| TEXAS INSTRUMENTS INCORPORATED
| Standard Linear and Logic Group
| IBIS Model of SN74CBTLV3253
| LOW-VOLTAGE DUAL 1-OF-4 FET MULTIPLEXER/DEMULTIPLEXER
| This file contains package information for the following:
|  SOIC 16-pin (D) package as [Component] CBTLV3253_D
|  TSSOP 16-pin (PW) package as [Component] CBTLV3253_PW
|  SSOP 16-pin (DBQR) package as [Component] CBTLV3253_DBQR
|  TVSOP 16-pin (DGV) package as [Component] CBTLV3253_DGV
|  QFN 16-pin (RGY) package as [Component] CBTLV3253_RGY
| This device can be powered at the following Vccs:
|  3.3 volt Vcc
|  2.5 volt Vcc
| This file provides unique models under the [Model Selector] for each Vcc.
| For operation at a specific Vcc, select the appropriate model after each
| [Model Selector] keyword.
[IBIS Ver]   3.2
[Comment char]  |_char
[File Name]   sn74cbtlv3253.ibs
[File Rev]   1.1 | x_die
[Date]   August 14, 2003
[Source]   Data created from TI-SPICE simulations at TI-SLL.
[Notes]   The following is an IBIS list for the CBTLV3253.
   Please contact sllibis@ti.com with questions and
   comments concerning SLL IBIS models.
   - The terminator models are for A-port only.
   - C_comp values have been replaced by the data sheet values in
   the terminator models.
   - Power clamp data deleted as there is no power-clamp diode.
   - Non-monotonic data due to FET characteristics.
[Disclaimer] Property of Texas Instruments Incorporated.  Unauthorized
   reproduction and/or distribution is strictly prohibited.
   This product is protected under copyright law.
   Created  2003, (C) Copyright  2003, Texas Instruments
   Incorporated, All Rights Reserved
   UNLESS THERE IS A SIGNED, WRITTEN AGREEMENT TO THE
   CONTRARY, TEXAS INSTRUMENTS (TI) IS PROVIDING THE IBIS
   MODELS  AND WITHOUT ANY WARRANTY, EXPRESSED OR
   IMPLIED.  TI assumes no liability for:
   1) the accuracy of the IBIS models provided to your
   company;
   2) the proper functioning of these IBIS Models in your
   design or for any resulting applications; or
   3) infringement of patents, copyrights or intellectual
   property rights resulting from your use of these IBIS
   models.
   TI provides IBIS Models as a service to our customers.
   You and your company shall not distribute, sell or give
   these models to anyone else without prior written
   permission from TI.
   TI reserves the right to make changes to our products or
   to discontinue any semiconductor product or service
   without notice, and advises our customers to obtain the
   latest version of relevant information to verify, before
   placing orders, that the information being relied on is
   current.
   Please be aware that your receipt and use of the IBIS
   information provided shall serve as acceptance of these
   terms and conditions.  If you do not accept these terms,
   you should return or destroy the IBIS models and any
   other accompanying information immediately.
| Component CBTLV3253_D 16-pin SOIC
[Component]   CBTLV3253_D
[Manufacturer]   Texas Instruments, Inc.
[Package]
|   typ   min   max
R_pkg   3.900e-02   2.800e-02   4.900e-02
L_pkg   3.453e-09   2.350e-09   4.375e-09
C_pkg   5.210e-13   2.540e-13   7.080e-13
[Pin]   signal_name   model_name   R_pin   L_pin   C_pin
1   1NOE   CBTLV3253_NOE   4.200e-02   4.336e-09   7.030e-13
2   S1   CBTLV3253_IN   4.900e-02   3.778e-09   6.340e-13
3   1B4   CBTLV3253_IO   2.800e-02   3.449e-09   5.180e-13
4   1B3   CBTLV3253_IO   2.900e-02   2.393e-09   2.540e-13
5   1B2   CBTLV3253_IO   2.800e-02   2.350e-09   2.640e-13
6   1B1   CBTLV3253_IO   4.800e-02   3.312e-09   4.830e-13
7   1A   CBTLV3253_IO   4.300e-02   3.629e-09   6.040e-13
8   GND   GND   4.400e-02   4.375e-09   7.080e-13
9   2A   CBTLV3253_IO   4.200e-02   4.336e-09   7.030e-13
10   2B1   CBTLV3253_IO   4.900e-02   3.778e-09   6.340e-13
11   2B2   CBTLV3253_IO   2.800e-02   3.449e-09   5.180e-13
12   2B3   CBTLV3253_IO   2.900e-02   2.393e-09   2.550e-13
13   2B4   CBTLV3253_IO   2.800e-02   2.350e-09   2.640e-13
14   S0   CBTLV3253_IN   4.800e-02   3.312e-09   4.830e-13
15   2NOE   CBTLV3253_NOE   4.300e-02   3.629e-09   6.040e-13
16   VCC   POWER   4.400e-02   4.375e-09   7.080e-13
| Component CBTLV3253_PW 16-pin TSSOP
[Component]   CBTLV3253_PW
[Manufacturer]   Texas Instruments, Inc.
[Package]
|   typ   min   max
R_pkg   4.500e-02   3.800e-02   5.100e-02
L_pkg   2.593e-09   2.447e-09   3.080e-09
C_pkg   2.810e-13   2.430e-13   3.770e-13
[Pin]   signal_name   model_name   R_pin   L_pin   C_pin
1   1NOE   CBTLV3253_NOE   4.000e-02   3.080e-09   3.770e-13
2   S1   CBTLV3253_IN   3.800e-02   2.458e-09   2.810e-13
3   1B4   CBTLV3253_IO   5.100e-02   2.512e-09   2.550e-13
4   1B3   CBTLV3253_IO   5.100e-02   2.447e-09   2.430e-13
5   1B2   CBTLV3253_IO   5.100e-02   2.447e-09   2.430e-13
6   1B1   CBTLV3253_IO   5.100e-02   2.512e-09   2.550e-13
7   1A   CBTLV3253_IO   3.800e-02   2.458e-09   2.810e-13
8   GND   GND   4.000e-02   3.080e-09   3.770e-13
9   2A   CBTLV3253_IO   3.900e-02   2.832e-09   3.160e-13
10   2B1   CBTLV3253_IO   3.800e-02   2.460e-09   2.790e-13
11   2B2   CBTLV3253_IO   5.100e-02   2.512e-09   2.550e-13
12   2B3   CBTLV3253_IO   5.100e-02   2.447e-09   2.430e-13
13   2B4   CBTLV3253_IO   5.100e-02   2.447e-09   2.430e-13
14   S0   CBTLV3253_IN   5.100e-02   2.512e-09   2.550e-13
15   2NOE   CBTLV3253_NOE   3.800e-02   2.459e-09   2.790e-13
16   VCC   POWER   3.900e-02   2.832e-09   3.160e-13
| Component CBTLV3253_DBQR 16-pin SSOP
[Component]   CBTLV3253_DBQR
[Manufacturer]   Texas Instruments, Inc.
[Package]
|   typ   min   max
R_pkg   3.800e-02   2.700e-02   5.900e-02
L_pkg   2.353e-09   1.491e-09   4.500e-09
C_pkg   2.100e-13   6.400e-14   5.920e-13
[Pin]   signal_name   model_name   R_pin   L_pin   C_pin
1   1NOE   CBTLV3253_NOE   5.800e-02   4.450e-09   5.920e-13
2   S1   CBTLV3253_IN   4.000e-02   1.930e-09   1.110e-13
3   1B4   CBTLV3253_IO   2.800e-02   1.538e-09   7.600e-14
4   1B3   CBTLV3253_IO   2.700e-02   1.491e-09   6.400e-14
5   1B2   CBTLV3253_IO   2.700e-02   1.491e-09   6.400e-14
6   1B1   CBTLV3253_IO   2.700e-02   1.506e-09   7.500e-14
7   1A   CBTLV3253_IO   3.300e-02   1.922e-09   1.090e-13
8   GND   GND   5.900e-02   4.500e-09   5.880e-13
9   2A   CBTLV3253_IO   5.800e-02   3.695e-09   4.140e-13
10   2B1   CBTLV3253_IO   3.400e-02   2.685e-09   2.820e-13
11   2B2   CBTLV3253_IO   2.900e-02   1.552e-09   7.700e-14
12   2B3   CBTLV3253_IO   2.800e-02   1.506e-09   6.500e-14
13   2B4   CBTLV3253_IO   2.700e-02   1.492e-09   6.400e-14
14   S0   CBTLV3253_IN   2.800e-02   1.534e-09   7.600e-14
15   2NOE   CBTLV3253_NOE   4.000e-02   2.703e-09   2.840e-13
16   VCC   POWER   5.600e-02   3.645e-09   4.180e-13
| Component CBTLV3253_DGV 16-pin TVSOP
[Component]   CBTLV3253_DGV
[Manufacturer]   Texas Instruments, Inc.
[Package]
|   typ   min   max
R_pkg   3.900e-02   3.300e-02   4.500e-02
L_pkg   2.543e-09   2.320e-09   2.938e-09
C_pkg   3.860e-13   3.340e-13   4.490e-13
[Pin]   signal_name   model_name   R_pin   L_pin   C_pin
1   1NOE   CBTLV3253_NOE   3.500e-02   2.907e-09   4.170e-13
2   S1   CBTLV3253_IN   4.200e-02   2.558e-09   4.460e-13
3   1B4   CBTLV3253_IO   3.800e-02   2.341e-09   3.450e-13
4   1B3   CBTLV3253_IO   3.800e-02   2.320e-09   3.340e-13
5   1B2   CBTLV3253_IO   3.900e-02   2.322e-09   3.340e-13
6   1B1   CBTLV3253_IO   3.800e-02   2.353e-09   3.420e-13
7   1A   CBTLV3253_IO   4.000e-02   2.536e-09   4.410e-13
8   GND   GND   3.300e-02   2.897e-09   4.180e-13
9   2A   CBTLV3253_IO   3.500e-02   2.927e-09   4.190e-13
10   2B1   CBTLV3253_IO   4.500e-02   2.632e-09   4.490e-13
11   2B2   CBTLV3253_IO   3.900e-02   2.368e-09   3.470e-13
12   2B3   CBTLV3253_IO   3.900e-02   2.330e-09   3.350e-13
13   2B4   CBTLV3253_IO   3.900e-02   2.320e-09   3.350e-13
14   S0   CBTLV3253_IN   3.900e-02   2.361e-09   3.450e-13
15   2NOE   CBTLV3253_NOE   4.100e-02   2.573e-09   4.460e-13
16   VCC   POWER   3.500e-02   2.938e-09   4.200e-13
| Component CBTLV3253_RGY 16-pin QFN
[Component]   CBTLV3253_RGY
[Manufacturer]   Texas Instruments, Inc.
[Package]
|   typ   min   max
R_pkg   3.000e-02   2.700e-02   3.800e-02
L_pkg   8.000e-10   7.220e-10   9.400e-10
C_pkg   1.410e-13   1.290e-13   1.550e-13
[Pin]   signal_name   model_name   R_pin   L_pin   C_pin
1   1NOE   CBTLV3253_NOE   2.700e-02   8.180e-10   1.320e-13
2   S1   CBTLV3253_IN   2.700e-02   8.030e-10   1.300e-13
3   1B4   CBTLV3253_IO   3.700e-02   9.080e-10   1.500e-13
4   1B3   CBTLV3253_IO   2.900e-02   7.220e-10   1.390e-13
5   1B2   CBTLV3253_IO   2.900e-02   7.220e-10   1.390e-13
6   1B1   CBTLV3253_IO   2.900e-02   7.300e-10   1.400e-13
7   1A   CBTLV3253_IO   2.900e-02   7.240e-10   1.390e-13
8   GND   GND   3.100e-02   8.000e-10   1.400e-13
9   2A   CBTLV3253_IO   2.700e-02   8.110e-10   1.290e-13
10   2B1   CBTLV3253_IO   2.800e-02   7.840e-10   1.310e-13
11   2B2   CBTLV3253_IO   3.700e-02   9.150e-10   1.530e-13
12   2B3   CBTLV3253_IO   2.900e-02   8.470e-10   1.520e-13
13   2B4   CBTLV3253_IO   2.900e-02   7.580e-10   1.430e-13
14   S0   CBTLV3253_IN   2.900e-02   7.720e-10   1.440e-13
15   2NOE   CBTLV3253_NOE   2.900e-02   7.400e-10   1.420e-13
16   VCC   POWER   3.800e-02   9.400e-10   1.550e-13
[Series Switch Groups]
| Function Group States
On  1 /   | 1A->1B1 NOE1 LOW, S1 LOW, S0 LOW
On  2 /   | 1A->1B2 NOE1 LOW, S1 LOW, S0 HIGH
On  3 /   | 1A->1B3 NOE1 LOW, S1 HIGH, S0 LOW
On  4 /   | 1A->1B4 NOE1 LOW, S1 HIGH, S0 HIGH
On  5 /   | 2A->2B1 NOE2 LOW, S1 LOW, S0 LOW
On  6 /   | 2A->2B2 NOE2 LOW, S1 LOW, S0 HIGH
On  7 /   | 2A->2B3 NOE2 LOW, S1 HIGH, S0 LOW
On  8 /   | 2A->2B4 NOE2 LOW, S1 HIGH, S0 HIGH
On  1 5 /   | Enable 1 5
On  2 6 /   | Enable 2 6
On  3 7 /   | Enable 3 7
On  4 8 /   | Enable 4 8
Off 1 2 3 4 5 6 7 8 /  | Disable All
[Series Pin Mapping]   pin_2   model_name   function_table_group
7   6   CBTLV3253_IO_33_S   1
| 7   6   CBTLV3253_IO_25_S   1
7   5   CBTLV3253_IO_33_S   2
| 7   5   CBTLV3253_IO_25_S   2
7   4   CBTLV3253_IO_33_S   3
| 7   4   CBTLV3253_IO_25_S   3
7   3   CBTLV3253_IO_33_S   4
| 7   3   CBTLV3253_IO_25_S   4
9   10   CBTLV3253_IO_33_S   5
| 9   10   CBTLV3253_IO_25_S   5
9   11   CBTLV3253_IO_33_S   6
| 9   11   CBTLV3253_IO_25_S   6
9   12   CBTLV3253_IO_33_S   7
| 9   12   CBTLV3253_IO_25_S   7
9   13   CBTLV3253_IO_33_S   8
| 9   13   CBTLV3253_IO_25_S   8
| Model CBTLV3253_NOE
[Model Selector]   CBTLV3253_NOE
CBTLV3253_NOE_33   3.3 volt Vcc
CBTLV3253_NOE_25   2.5 volt Vcc
| Model CBTLV3253_IN
[Model Selector]   CBTLV3253_IN
CBTLV3253_IN_33   3.3 volt Vcc
CBTLV3253_IN_25   2.5 volt Vcc
| Model CBTLV3253_IO
[Model Selector]   CBTLV3253_IO
CBTLV3253_IO_33   3.3 volt Vcc
CBTLV3253_IO_25   2.5 volt Vcc
| Model CBTLV3253_IO_S
[Model Selector]   CBTLV3253_IO_S
CBTLV3253_IO_33_S   3.3 volt Vcc_S
CBTLV3253_IO_25_S   2.5 volt Vcc_S
[Model]   CBTLV3253_IO_33_S
Model_type  Series_switch
| variable   typ   min   max
C_comp   0   0   0
[Temperature Range]   40   100   -40
| Ambient temperature   25   85   -40
[Voltage range]   3.3   3   3.6
[On]
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[Off]
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[Model]   CBTLV3253_IO_25_S
Model_type  Series_switch
| variable   typ   min   max
C_comp   0   0   0
[Temperature Range]   40   100   -40
| Ambient temperature   25   85   -40
[Voltage range]   2.5   2.3   2.7
[On]
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[Off]
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| Models and submodels in the file (8): CBTLV3253_NOE_33 (Input), CBTLV3253_NOE_25 (Input), CBTLV3253_IN_33 (Input), CBTLV3253_IN_25 (Input), CBTLV3253_IO_33_S (Series_switch), CBTLV3253_IO_33 (Terminator), CBTLV3253_IO_25_S (Series_switch), CBTLV3253_IO_25 (Terminator)
